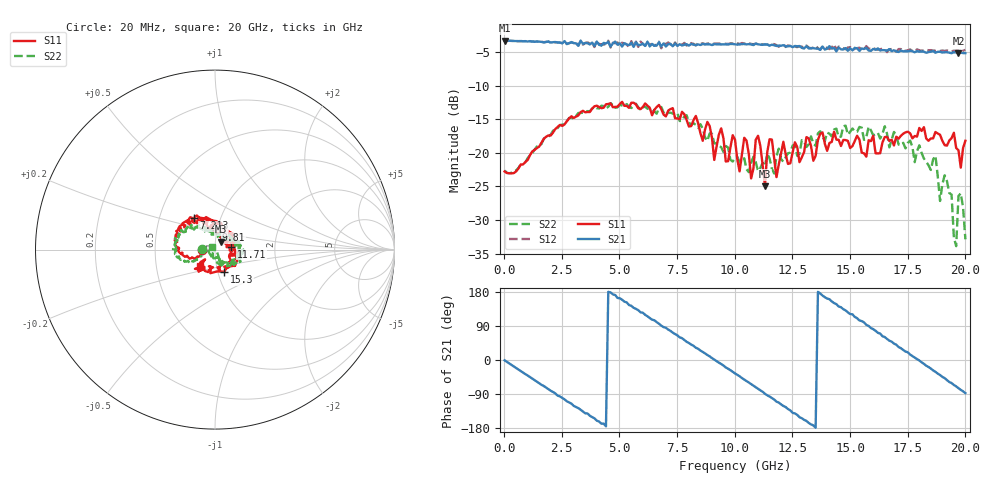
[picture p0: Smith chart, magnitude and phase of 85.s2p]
!Agilent Technologies,N5230A,US43500223,A.07.50.48
!Agilent N5230A: A.07.50.48
!Date: Sunday, September 13, 2015 20:56:50
!Correction: S11(Full 2 Port(1,2))
!S21(Full 2 Port(1,2))
!S12(Full 2 Port(1,2))
!S22(Full 2 Port(1,2))
!S2P File: Measurements: S11, S21, S12, S22:
# Hz S  dB  R 50
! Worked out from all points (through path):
!   201 points, 20 MHz to 20 GHz, reference 50 ohm
!   highest |S21| = -3.29 dB at 20 MHz (marker M1); lowest = -5.2 dB at 19.7 GHz (marker M2)
!   group delay of S21, straight-line fit = 112 ps
!   lowest |S11| = -25.0 dB at 11.31 GHz (marker M3), VSWR 1.12, Z = 53.4 + j4.77 ohm
!   |S11| at or under -10 dB: start of sweep to end of sweep
!   |S22| runs from -33.9 to -12.6 dB; largest |S21 - S12| = 0.051
!   S11 on the Smith chart (normalised r, x): 20 MHz: 0.86, +0.00; 7.213 GHz: 0.74, +0.27; 9.81 GHz: 0.99, +0.22; 11.71 GHz: 1.20, +0.04; 15.3 GHz: 1.07, -0.27; 20 GHz: 0.83, -0.16
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2e7  -22.77 179.7  -3.29 -0.9  -3.29 -0.9  -22.63 179.2
1.9181e9  -17.42 -161.3  -3.43 -76.9  -3.46 -77.1  -17.60 -151.1
3.4166e9  -13.75 -178.1  -3.76 -136.0  -3.92 -137.9  -14.03 -163.4
4.8152e9  -13.16 158.2  -3.45 171.6  -3.69 172.8  -13.30 179.4
6.7133e9  -12.88 127.4  -3.55 95.8  -3.47 95.2  -13.34 151.1
7.2128e9  -13.49 124.4  -3.79 76.8  -3.86 75.5  -14.03 141.3
9.8102e9  -19.23 87.6  -3.81 -26.9  -3.69 -27.9  -21.04 99.7
1.001e10  -18.04 54.8  -3.86 -35.4  -3.77 -36.2  -20.73 96.2
1.07093e10  -23.81 46.7  -3.87 -63.6  -3.79 -65.5  -21.50 76.9
1.1009e10  -17.46 41.2  -3.86 -76.3  -3.86 -78.1  -22.72 78.5
1.13087e10  -24.98 52.2  -3.87 -89.1  -3.88 -90.5  -21.96 56.9
1.15085e10  -17.99 41.8  -4.06 -96.4  -3.99 -99.0  -20.81 59.1
1.17083e10  -20.83 10.7  -4.00 -104.2  -3.83 -106.0  -23.07 41.3
1.34066e10  -21.18 -26.4  -4.44 -172.6  -4.32 -172.6  -18.63 10.3
1.53047e10  -17.46 -67.1  -4.46 110.3  -4.42 110.3  -16.87 -8.0
1.67033e10  -18.25 -119.0  -4.57 51.0  -4.60 50.7  -19.18 -32.4
1.87013e10  -16.90 -125.4  -5.10 -31.2  -4.82 -33.6  -20.43 -69.0
1.89011e10  -17.31 -130.6  -4.97 -39.7  -4.86 -43.6  -27.16 -78.4
1.94006e10  -17.82 -128.0  -5.18 -60.8  -4.90 -64.8  -26.22 -101.6
1.96004e10  -19.28 -139.1  -5.07 -69.7  -4.82 -72.9  -33.89 -52.3
1.97003e10  -19.62 -139.0  -5.19 -74.5  -4.82 -79.1  -26.41 -63.7
2e10  -18.20 -132.0  -5.17 -87.4  -4.69 -91.2  -32.86 137.7
